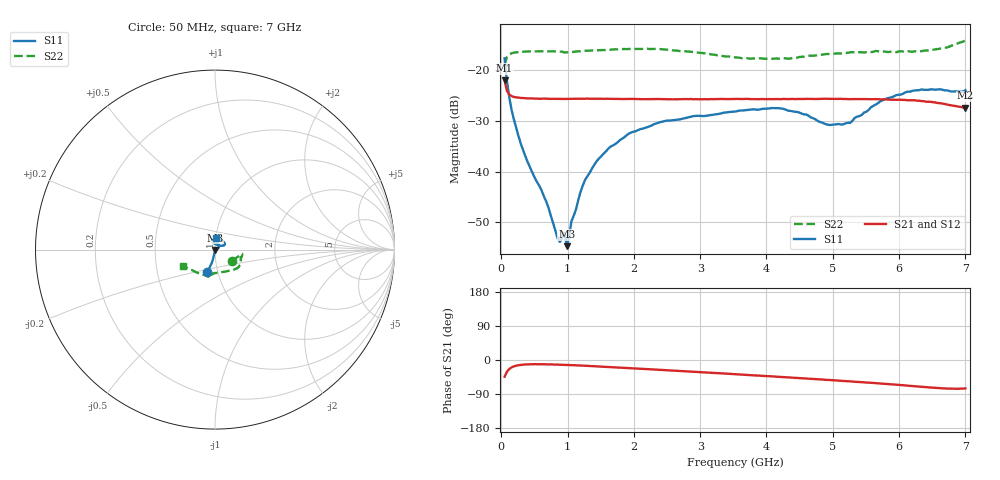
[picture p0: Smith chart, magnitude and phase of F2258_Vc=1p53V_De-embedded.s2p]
! Integrated Device Technology
! Corporate Headquarters
! 6024 Silver Creek Valley Road
! San Jose, CA 95138  USA
! Phone:  1-408-284-8200
! Toll Free:  1-800-223-1366
! Webpage:  http://www.idt.com/
! Timing and RF Division
! 515 Groton Road, Suite 102
! Westford, MA 01886-6024
! Device:  F2258
! Description: Voltage Variable RF Attenuator
! Frequency:  50.0 -  6000.00 MHz
! Package:  3x3 mm Thin QFN Plastic Package: 16 pin
! Ports:  2 RF, 2 DC
!  Pin  1  = NC
!  Pin  2  = NC
!  Pin  3  = RF2  = Port 2
!  Pin  4  = GND
!  Pin  5  = Vdd
!  Pin  6  = NC
!  Pin  7  = VCTRL
!  Pin  8  = NC
!  Pin  9  = GND
!  Pin 10  = RF1  = Port 1
!  Pin 11  = NC
!  Pin 12  = NC
!  Pin 13  = NC
!  Pin 14  = NC
!  Pin 15  = NC
!  Pin 16  = NC
! Vcntrl:  1.530 Volts
! Vdd:  +3.300 Volts
! Current:  1.162 mA
! Data:  The device was measured on a the F2258 evaluation board which has
!  individual transmission lines to the RF pins.  Data was collected
!  using a calibrated network analyzer.  The evaluation board was
!  de-embedded using a TRL calibration technique.
!  The reference plane is the edge of the package pin.
! Misc:  SN 10
!  Action Tracker AT0285
! Date Measured:  2014-12-10
! Date:  2016-01-13  MJV
! Note:
!  Integrated Device Technology supplies this data as a sample of measured
!  data at the package pin for this product.  Your particular data for this
!  product may vary.
!  Data was taken at 25 degrees C.
!  Integrated Device Technology reserves the right to change this data at anytime.
!Freq_(GHz)  S11M_(dB)  S11P_(deg)  S21M_(dB)  S21P_(deg)  S12M_(dB)  S12P_(deg)  S22M_(dB)  S22P_(deg)
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# GHz S dB R 50
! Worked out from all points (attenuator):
!   201 points, 50 MHz to 7 GHz, reference 50 ohm
!   highest |S21| = -21.98 dB at 50 MHz (marker M1); lowest = -27.4 dB at 7 GHz (marker M2)
!   lowest |S11| = -54.8 dB at 988.2 MHz (marker M3), VSWR 1.00, Z = 50.1 - j0.17 ohm
!   |S11| at or under -10 dB: start of sweep to end of sweep
!   |S22| runs from -18.9 to -14.1 dB; largest |S21 - S12| = 0.00049
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0.05  -17.60 -108.6  -21.98 -44.0  -21.93 -43.9  -18.90 -33.4
0.08475  -22.07 -104.0  -24.04 -31.1  -24.00 -31.0  -17.34 -16.2
0.15425  -27.73 -101.7  -25.07 -19.6  -25.02 -19.6  -16.63 -10.0
0.29325  -34.44 -99.7  -25.44 -12.9  -25.42 -12.9  -16.33 -8.6
0.6755  -45.86 -81.2  -25.59 -11.4  -25.59 -11.4  -16.20 -12.8
0.84925  -53.18 -37.8  -25.64 -12.2  -25.61 -12.2  -16.27 -15.9
0.884  -53.91 -16.4  -25.62 -12.4  -25.60 -12.4  -16.29 -16.7
0.9535  -52.07 -81.3  -25.63 -12.8  -25.61 -12.8  -16.46 -17.3
0.98825  -54.75 -68.5  -25.63 -13.0  -25.63 -13.0  -16.43 -18.1
1.05775  -49.83 -13.6  -25.62 -13.5  -25.58 -13.5  -16.37 -19.3
1.2315  -42.69 11.7  -25.59 -14.9  -25.61 -14.9  -16.15 -22.0
1.44  -37.93 15.7  -25.61 -17.0  -25.59 -16.9  -16.05 -25.3
1.6485  -35.05 20.0  -25.63 -18.9  -25.61 -18.9  -15.90 -28.5
2.37825  -30.30 39.8  -25.66 -25.8  -25.67 -25.8  -15.80 -39.2
3.525  -28.14 87.7  -25.64 -37.4  -25.64 -37.4  -17.42 -66.0
4.22  -27.52 103.9  -25.69 -44.8  -25.67 -44.8  -17.69 -88.1
4.7065  -29.47 93.7  -25.64 -50.0  -25.62 -50.0  -17.11 -97.5
4.94975  -30.79 76.6  -25.65 -52.7  -25.63 -52.8  -16.76 -100.3
5.2625  -30.37 48.5  -25.67 -56.3  -25.64 -56.4  -16.43 -102.5
5.85325  -25.43 26.0  -25.78 -63.9  -25.72 -63.9  -16.35 -105.9
6.33975  -23.76 32.3  -26.07 -70.8  -26.06 -70.8  -16.20 -117.4
7  -23.91 83.5  -27.36 -75.0  -27.35 -75.0  -14.08 -153.2
